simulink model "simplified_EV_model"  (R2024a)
settings: Solver=VariableStepAuto  StartTime=0.0  StopTime=t_sim  RelTol=1e-6
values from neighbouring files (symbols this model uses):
  A_f = 2.15    [main.m]    (also in prediction_longitudinal_model.m; MPC_and_plant_params.m; prediction_model_test.m; main_BW_FW.m)
  alpha = 0*pi/180    (= 0)    [main.m]    (also in prediction_longitudinal_model.m; MPC_and_plant_params.m; prediction_model_test.m; main_BW_FW.m)
  C_d = 0.33    [main.m]    (also in prediction_longitudinal_model.m; MPC_and_plant_params.m; prediction_model_test.m; main_BW_FW.m)
  f_0 = 4.5*1e-3    (= 0.0045)    [main.m]    (also in prediction_longitudinal_model.m; MPC_and_plant_params.m; prediction_model_test.m; main_BW_FW.m)
  g = 9.81    [main.m]    (also in prediction_longitudinal_model.m; MPC_and_plant_params.m; prediction_model_test.m; main_BW_FW.m)
  k = 0    [main.m]    (also in prediction_longitudinal_model.m; MPC_and_plant_params.m; prediction_model_test.m; main_BW_FW.m)
  M_veh = 1400    [main.m]    (also in prediction_longitudinal_model.m; MPC_and_plant_params.m; prediction_model_test.m; main_BW_FW.m)
  N_p = 1    [main.m]    (also in prediction_longitudinal_model.m; MPC_and_plant_params.m; prediction_model_test.m; main_BW_FW.m)
  N_s = 108    [main.m]    (also in prediction_longitudinal_model.m; MPC_and_plant_params.m; prediction_model_test.m; main_BW_FW.m)
  r_w = 0.3    [main.m]    (also in prediction_longitudinal_model.m; MPC_and_plant_params.m; prediction_model_test.m; main_BW_FW.m)
  rho = 1.25    [main.m]    (also in prediction_longitudinal_model.m; MPC_and_plant_params.m; prediction_model_test.m; main_BW_FW.m)
  Ro_s = F_Ro_s(SOC_vec)    [main.m]    (also in MPC_and_plant_params.m; main_BW_FW.m)
  s = tf('s')    [main.m]    (also in MPC_and_plant_params.m; polinomial_fits.m = size(Speed))
  SOC0 = 0.8    [main.m]    (also in MPC_and_plant_params.m; prediction_model_test.m; main_BW_FW.m)
  SOC_vec = linspace(0,1,500)    [main.m]    (also in MPC_and_plant_params.m; main_BW_FW.m)
  tau_gb = 9.6    [main.m]    (also in prediction_longitudinal_model.m; MPC_and_plant_params.m; prediction_model_test.m; main_BW_FW.m)
  Voc_s = F_Voc_s(SOC_vec)    [main.m]    (also in MPC_and_plant_params.m; main_BW_FW.m)
undefined symbols (not defined in the file or in its folder): Efficiency, flip, m, seconds, Shaft_Torque, Speed
libraries: autolibshared x1

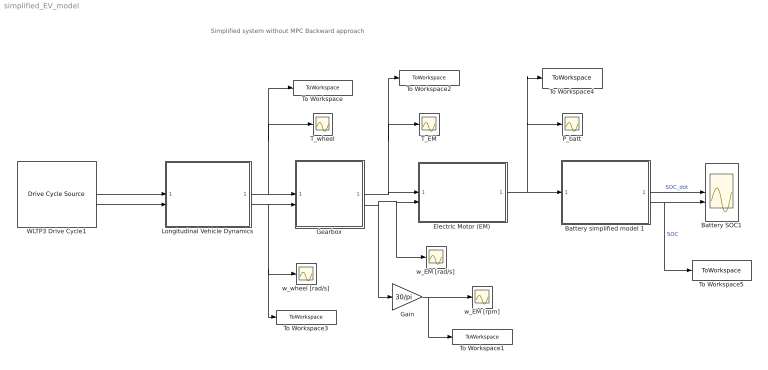
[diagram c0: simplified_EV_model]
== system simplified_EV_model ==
  note: Simplified system without MPC Backward approach
  Battery SOC1 : Scope  NumInputPorts=2
  Battery simplified model 1 : Subsystem
  Electric Motor (EM) : Subsystem
  Gain : Gain  Gain=30/pi
  Gearbox : Subsystem
  Longitudinal Vehicle Dynamics : Subsystem
  P_batt : Scope
  T_EM : Scope
  T_wheel : Scope
  To Workspace : ToWorkspace  VariableName=T_wheel  SaveFormat=Timeseries  SampleTime=-1
  To Workspace1 : ToWorkspace  VariableName=w_EM_rpm  SaveFormat=Timeseries  SampleTime=-1
  To Workspace2 : ToWorkspace  VariableName=T_EM  SaveFormat=Timeseries  SampleTime=-1
  To Workspace3 : ToWorkspace  VariableName=w_wheel  SaveFormat=Timeseries  SampleTime=-1
  To Workspace4 : ToWorkspace  VariableName=P_batt  SaveFormat=Timeseries  SampleTime=-1
  To Workspace5 : ToWorkspace  VariableName=SOC  SaveFormat=Timeseries  SampleTime=-1
  WLTP3 Drive Cycle1 : autolibshared/Drive Cycle Source  cycleVar=Workspace variable  wsVar=vehspeed  fileVar=cycleFTP75.mat  tfinal="1800  seconds"  cycleRepeat=off  outAccPort=on  outGearPort=off  gearList=No gear data  t_wot1=5  xdot_woto=0  xdot_wot1=30  t_wot2=20  xdot_wot2=0  t_wotend=30  srcUnit=m/s  outUnit=m/s  srcAccUnit=m/s/s  outAccUnit=m/s^2  dt=0  aMode=1  faultOption=off  velBnd=2  velBndUnit=mph  inUnit=m/s  timeBnd=1  failOption=off  stopSim=off  maxFaultCnt=10  maxFaultTime=2  maxTotFaultTime=15  traceOption=off  dtTrace=1  traceWindow=10  lastDCname=Custom Data Set  lastOutUnit=mph  lastDT=0  lastTB=1  lastSB=2  forceCalcBound=off
  w_EM [rad/s] : Scope
  w_EM [rpm] : Scope
  w_wheel [rad/s] : Scope
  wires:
  Electric Motor (EM)/1(P_batt) -> Battery simplified model 1/1(P_batt), To Workspace4/1, P_batt/1
  Battery simplified model 1/1(SOC_dot) -> Battery SOC1/1  "SOC_dot"
  Battery simplified model 1/2(SOC) -> To Workspace5/1, Battery SOC1/2  "SOC"
  Longitudinal Vehicle Dynamics/1(T_wheel) -> Gearbox/1(T_wheel), To Workspace/1, T_wheel/1
  Longitudinal Vehicle Dynamics/2(w_wheel) -> Gearbox/2(w_wheel), To Workspace3/1, w_wheel [rad/s]/1
  Gearbox/1(T_EM) -> To Workspace2/1, T_EM/1, Electric Motor (EM)/1(T_EM)
  Gearbox/2(w_EM) -> w_EM [rad/s]/1, Electric Motor (EM)/2(w_EM), Gain/1
  Gain/1 -> To Workspace1/1, w_EM [rpm]/1
  WLTP3 Drive Cycle1/1 -> Longitudinal Vehicle Dynamics/1(v_ref)
  WLTP3 Drive Cycle1/2 -> Longitudinal Vehicle Dynamics/2(a_ref)

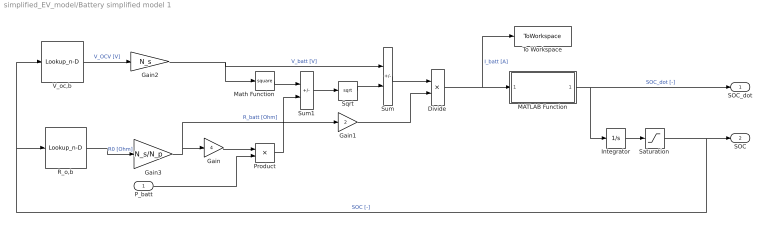
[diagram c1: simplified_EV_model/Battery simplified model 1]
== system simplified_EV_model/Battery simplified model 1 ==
  P_batt : Inport
  Divide : Product  Inputs=*/
  Gain : Gain  Gain=4
  Gain1 : Gain  Gain=2
  Gain2 : Gain  Gain=N_s
  Gain3 : Gain  Gain=N_s/N_p
  Integrator : Integrator  InitialCondition=SOC0
  MATLAB Function : MATLAB Function  TreatAsAtomicUnit=on
  Math Function : Math  Operator=square
  Product : Product
  R_o,b : Lookup_n-D  NumberOfTableDimensions=1  BreakpointsForDimension1=SOC_vec  BreakpointsForDimension3=[5, 7]  Table=Ro_s  InternalRulePriority=Speed  RndMeth=Simplest
  Saturation : Saturate  UpperLimit=1  LowerLimit=0
  Sqrt : Sqrt
  Sum : Sum  Inputs=+-
  Sum1 : Sum  Inputs=+-
  To Workspace : ToWorkspace  VariableName=Ib  SaveFormat=Timeseries  SampleTime=-1
  V_oc,b : Lookup_n-D  NumberOfTableDimensions=1  BreakpointsForDimension1=SOC_vec  BreakpointsForDimension3=[5, 7]  Table=Voc_s  InternalRulePriority=Speed  RndMeth=Simplest
  SOC_dot : Outport
  SOC : Outport  Port=2
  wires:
  Integrator/1 -> Saturation/1
  R_o,b/1 -> Gain3/1  "R0 [Ohm]"
  MATLAB Function/1(SOC_dot) -> SOC_dot/1, Integrator/1  "SOC_dot [-]"
  Gain2/1 -> Sum/1, Math Function/1  "V_batt [V]"
  Divide/1 -> MATLAB Function/1(I_b), To Workspace/1  "I_batt [A]"
  Sum1/1 -> Sqrt/1
  Sum/1 -> Divide/1
  Sqrt/1 -> Sum/2
  Gain1/1 -> Divide/2
  Saturation/1 -> R_o,b/1, V_oc,b/1, SOC/1  "SOC [-]"
  Math Function/1 -> Sum1/1
  Product/1 -> Sum1/2
  P_batt/1 -> Product/2
  V_oc,b/1 -> Gain2/1  "V_OCV [V]"
  Gain3/1 -> Gain1/1, Gain/1  "R_batt [Ohm]"
  Gain/1 -> Product/1

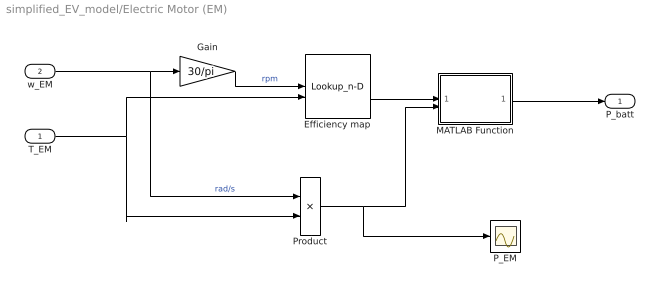
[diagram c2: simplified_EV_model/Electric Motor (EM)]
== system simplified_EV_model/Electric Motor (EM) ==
  T_EM : Inport
  w_EM : Inport  Port=2
  Efficiency map : Lookup_n-D  BreakpointsForDimension1=Speed(:,1)  BreakpointsForDimension2=flip(Shaft_Torque(1,:))  BreakpointsForDimension3=[5, 7]  Table=flip(Efficiency,2)/100  InternalRulePriority=Speed  RndMeth=Simplest
  Gain : Gain  Gain=30/pi
  MATLAB Function : MATLAB Function  TreatAsAtomicUnit=on
  P_EM : Scope
  Product : Product
  P_batt : Outport
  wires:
  w_EM/1 -> Product/1, Gain/1  "rad/s"
  T_EM/1 -> Efficiency map/2, Product/2
  Product/1 -> P_EM/1, MATLAB Function/2(P_EM)
  MATLAB Function/1(P_batt) -> P_batt/1
  Efficiency map/1 -> MATLAB Function/1(eta_EM)
  Gain/1 -> Efficiency map/1  "rpm"

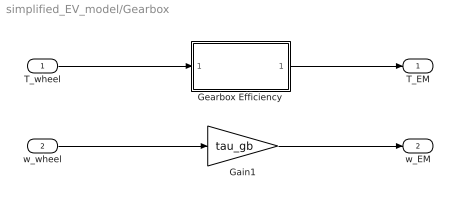
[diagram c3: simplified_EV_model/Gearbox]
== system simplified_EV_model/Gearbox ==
  T_wheel : Inport
  w_wheel : Inport  Port=2
  Gain1 : Gain  Gain=tau_gb
  Gearbox Efficiency : MATLAB Function  TreatAsAtomicUnit=on
  T_EM : Outport
  w_EM : Outport  Port=2
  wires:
  Gain1/1 -> w_EM/1
  Gearbox Efficiency/1(T_EM) -> T_EM/1
  T_wheel/1 -> Gearbox Efficiency/1(T_out)
  w_wheel/1 -> Gain1/1

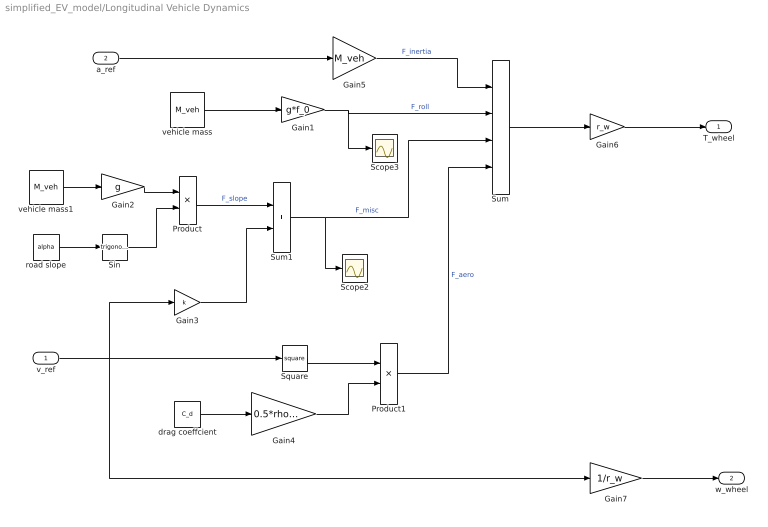
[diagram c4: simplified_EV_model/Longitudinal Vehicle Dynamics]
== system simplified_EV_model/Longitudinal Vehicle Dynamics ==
  v_ref : Inport
  a_ref : Inport  Port=2
  Gain1 : Gain  Gain=g*f_0
  Gain2 : Gain  Gain=g
  Gain3 : Gain  Gain=k
  Gain4 : Gain  Gain=0.5*rho*A_f
  Gain5 : Gain  Gain=M_veh
  Gain6 : Gain  Gain=r_w
  Gain7 : Gain  Gain=1/r_w
  Product : Product
  Product1 : Product
  Scope2 : Scope
  Scope3 : Scope
  Sin : Trigonometry
  Square : Math  Operator=square
  Sum : Sum  Inputs=++++
  Sum1 : Sum
  drag coeffcient : Constant  Value=C_d
  road slope : Constant  Value=alpha
  vehicle mass : Constant  Value=M_veh
  vehicle mass1 : Constant  Value=M_veh
  T_wheel : Outport
  w_wheel : Outport  Port=2
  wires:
  drag coeffcient/1 -> Gain4/1
  Gain4/1 -> Product1/2
  Sum1/1 -> Scope2/1, Sum/3  "F_misc"
  Gain2/1 -> Product/1
  vehicle mass/1 -> Gain1/1
  Gain1/1 -> Scope3/1, Sum/2  "F_roll"
  Square/1 -> Product1/1
  vehicle mass1/1 -> Gain2/1
  road slope/1 -> Sin/1
  Gain5/1 -> Sum/1  "F_inertia"
  Product1/1 -> Sum/4  "F_aero"
  Sin/1 -> Product/2
  Gain6/1 -> T_wheel/1
  Product/1 -> Sum1/1  "F_slope"
  Gain3/1 -> Sum1/2
  Sum/1 -> Gain6/1
  a_ref/1 -> Gain5/1
  v_ref/1 -> Gain3/1, Gain7/1, Square/1
  Gain7/1 -> w_wheel/1

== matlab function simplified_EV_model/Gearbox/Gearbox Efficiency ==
function T_EM = fcn(T_out)
eta_gb = 0.97;
tau_gb = 9.6;

T_EM = T_out/(tau_gb*eta_gb^(sign(T_out)));

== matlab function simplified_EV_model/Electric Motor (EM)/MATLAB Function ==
function P_batt = fcn(eta_EM,P_EM)
eta_inv = 1;

P_batt = P_EM/((eta_EM*eta_inv)^(sign(P_EM)));

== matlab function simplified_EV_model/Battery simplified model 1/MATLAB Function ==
function SOC_dot = fcn(I_b)
    eta_c = 0.95;
    Q_nom = 60*1*3600;
    if I_b > 0 % discharge
        SOC_dot = -I_b/(eta_c*Q_nom);
    else % charge
        SOC_dot = -eta_c*I_b/Q_nom;
    end
